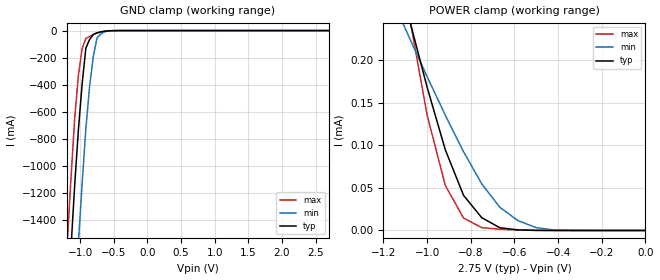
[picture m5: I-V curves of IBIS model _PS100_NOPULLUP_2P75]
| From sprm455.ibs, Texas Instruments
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|   Model Cell _PS100_NOPULLUP_2P75
|IDG09_PS100_NOPULLUP_2P75
[Model]   _PS100_NOPULLUP_2P75
Model_type   Input
Polarity   Non-Inverting
Vinl =  0.7V
Vinh =  1.7V
C_comp   1.261p   1.175p   1.435p
[Model Spec]
Vinl   0.7V   0.7V   0.7V
Vinh   1.7V   1.7V   1.7V
[Temperature Range]   25   125   -40
[Voltage Range]   2.75   2.5   3
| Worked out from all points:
|   GND clamp passes 1 mA (typ) near -0.54 V on its own axis
|   POWER clamp passes 1 mA (typ) near -1.78 V on its own axis
[POWER_clamp]
|   voltage   I(typ)   I(min)   I(max)
-2.75V    2.078mA    1.233mA    3.105mA
-1.111V   278.5uA    243.6uA    297.9uA
-1.083V   250uA      227.6uA    254.3uA
-1.056V   222.8uA    212uA      214.7uA
-1V       168.4uA    180.8uA    135.5uA
-916.7mV  94.71uA    135.4uA    52.81uA
-833.3mV  41.32uA    92.61uA    14.65uA
-750mV    15.05uA    54.85uA    3.347uA
-666.7mV  3.185uA    27.16uA    1.455uA
-583.3mV  666.6nA    11.53uA    482.3nA
-416.7mV  18.09nA    524.3nA    5.125nA
0V        50.28pA    7.906nA    617.3fA
[GND_clamp]
|   voltage   I(typ)   I(min)   I(max)
-2.75V    -17.11A    -17.95A    -16.64A
-1.194V   -2.105A    -3.008A    -1.577A
-1.139V   -1.621A    -2.516A    -1.105A
-1.083V   -1.151A    -2.031A    -653.7mA
-1.028V   -736.7mA   -1.572A    -333.3mA
-972.2mV  -396.6mA   -1.136A    -134.8mA
-916.7mV  -130.4mA   -725.1mA   -58.04mA
-861.1mV  -65.94mA   -415.2mA   -42.87mA
-805.6mV  -27.96mA   -191.3mA   -29.63mA
-750mV    -16.46mA   -53.27mA   -18.31mA
-638.9mV  -5.248mA   -9.009mA   -4.64mA
2.694V    49.16pA    10.7nA     439.6fA
